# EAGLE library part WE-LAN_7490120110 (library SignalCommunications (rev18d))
WE-LAN LAN Transformer 10/100 Base T - Compliant with IEEE 802.3, IEEE 802.3af and IEEE 802.3at standards - SMT -- Ethernet -- Power over Ethernet -- 1 Gigabit Ethernet -- Compliant with most IC's for ethernet applications like Intel, AMD, Globespan and Realtek -- Hub, Router, Switch Details see: http://katalog.we-online.de/en/pbs/WE-LAN/S 2016 (C) Würth Elektronik
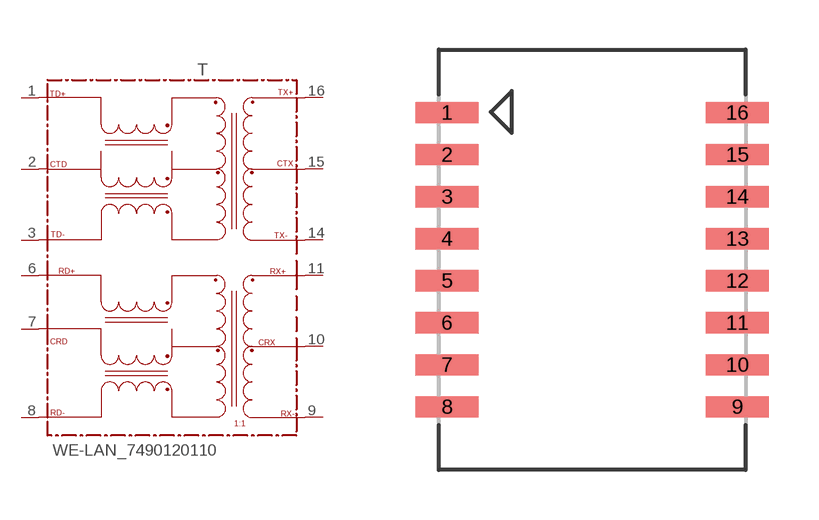
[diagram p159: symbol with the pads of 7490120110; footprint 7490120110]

Designator prefix T

## WE-LAN_7490120110  [7490120110]
1  1
2  2
3  3
6  6
7  7
8  8
9  9
10  10
11  11
14  14
15  15
16  16

## Footprint 7490120110 (pad centres in mm)
smd 1.91 x 0.64: 1 -4.385,4.445; 2 -4.385,3.175; 3 -4.385,1.905; 4 -4.385,0.635; 5 -4.385,-0.635; 6 -4.385,-1.905; 7 -4.385,-3.175; 8 -4.385,-4.445; 9 4.385,-4.445; 10 4.385,-3.175; 11 4.385,-1.905; 12 4.385,-0.635; 13 4.385,0.635; 14 4.385,1.905; 15 4.385,3.175; 16 4.385,4.445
